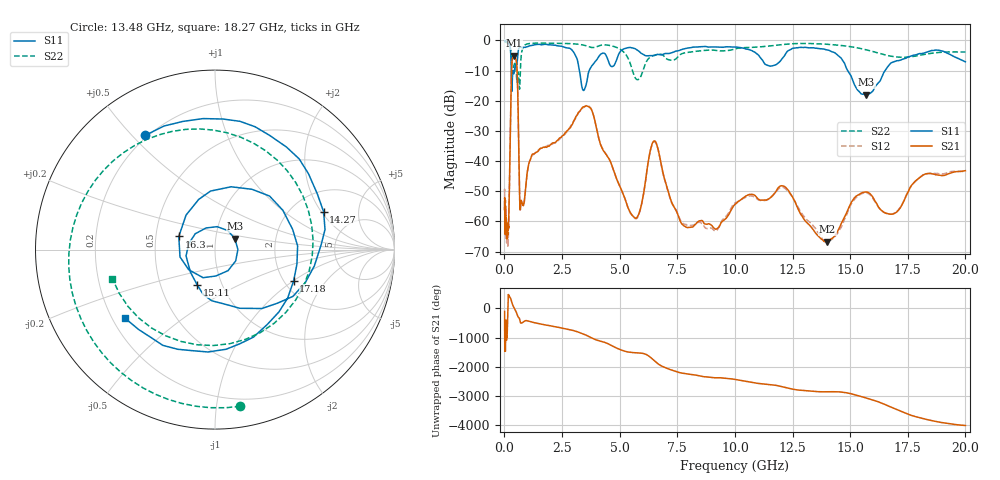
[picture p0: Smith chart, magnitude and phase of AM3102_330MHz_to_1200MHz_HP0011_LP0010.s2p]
! Date/Time: Tue, Sep 11, 2018 5:11 PM
! Network Analyzer: Agilent Technologies E8362B Rev: A.07.50.63
! Sweep from 0.010 to 20.000 GHz, 1601 Points, Sweep Type: LOG
! Power Supply: 4.950 V, 0.001 A
# Hz S DB R 50
!freq MagS11 AngS11 MagS21 AngS21 MagS12 AngS12 MagS22 AngS22
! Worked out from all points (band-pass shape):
!   1601 points, 10 MHz to 20 GHz, reference 50 ohm
!   highest |S21| = -5.05 dB at 410.6 MHz (marker M1); lowest = -66.8 dB at 14.01 GHz (marker M2)
!   |S21| within 3 dB of the highest: 322.6 MHz to 537.3 MHz (214.7 MHz wide, 49.9 % of centre)
!   lowest |S11| = -18.0 dB at 15.7 GHz (marker M3), VSWR 1.29, Z = 61.9 + j7.66 ohm
!   |S11| at or under -10 dB: 298.7 MHz to 364.9 MHz (66.2 MHz wide, 19.9 % of centre); 3.255 GHz to 3.677 GHz (422.6 MHz wide, 12.2 % of centre); 14.89 GHz to 16.51 GHz (1.62 GHz wide, 10.3 % of centre)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
!   |S22| runs from -16.2 to -0.2 dB; largest |S21 - S12| = 0.0083
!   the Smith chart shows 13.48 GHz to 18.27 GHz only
!   S11 on the Smith chart (normalised r, x): 13.48 GHz: 0.19, +0.55; 14.27 GHz: 2.95, +2.10; 15.11 GHz: 0.76, -0.31; 16.3 GHz: 0.66, +0.10; 17.18 GHz: 2.25, -1.01; 18.27 GHz: 0.25, -0.32
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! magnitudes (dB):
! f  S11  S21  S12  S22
! 10 MHz  0.0  -55.6  -50.6  -0.2
! 35.55 MHz  0.0  -58.6  -60.1  -0.4
! 126.4 MHz  -0.4  -62.1  -62.6  -0.8
! 169.7 MHz  -0.8  -62.7  -65.4  -1.1
! 410.6 MHz  -11.0  -5.1  -5.1  -8.5
! 447.2 MHz  -9.3  -5.4  -5.4  -7.6
! 559.1 MHz  -6.9  -11.2  -11.3  -13.5
! 685.8 MHz  -2.3  -56.2  -56.6  -12.2
! 1.59 GHz  -1.4  -35.7  -35.7  -0.9
! 3.651 GHz  -10.6  -21.9  -21.7  -2.0
! 5.652 GHz  -2.7  -58.7  -58.9  -12.1
! 6.518 GHz  -4.9  -33.3  -33.5  -4.9
! 7.882 GHz  -2.6  -61.9  -61.0  -4.0
! 13.48 GHz  -2.5  -63.7  -62.2  -1.1
! 14.01 GHz  -3.1  -66.8  -66.5  -1.3
! 14.27 GHz  -3.9  -65.3  -65.6  -1.4
! 15.11 GHz  -13.2  -53.0  -53.5  -2.2
! 15.7 GHz  -18.0  -50.3  -50.6  -3.1
! 16.3 GHz  -13.4  -56.0  -56.0  -4.3
! 17.18 GHz  -6.5  -55.5  -55.3  -5.6
! 18.27 GHz  -4.0  -44.2  -44.2  -4.5
! 20 GHz  -7.1  -43.2  -43.5  -3.8
